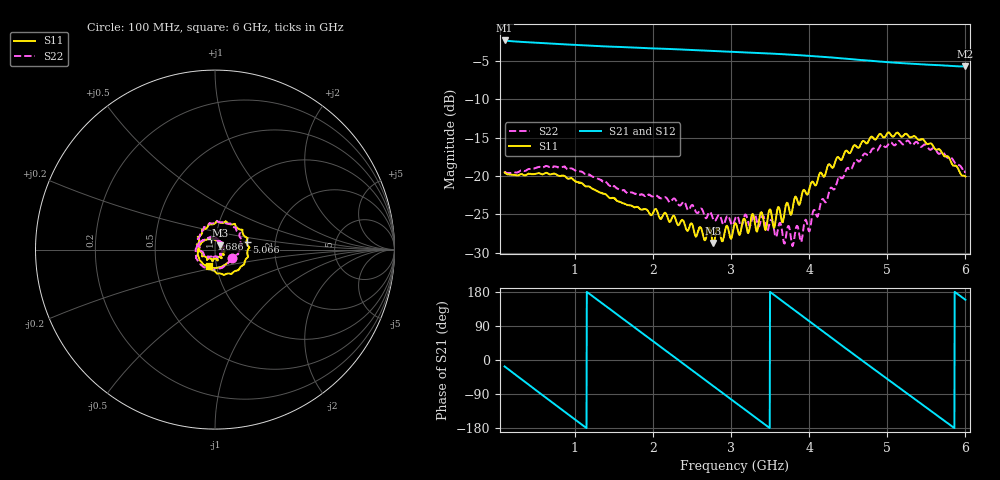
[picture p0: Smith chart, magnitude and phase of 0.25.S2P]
!Agilent Technologies,E5071C,MY46316741,A.11.02
!Date: Thu Dec 16 09:44:38 2021
!Data & Calibration Information:
!Freq	S11:SOLT4(ON)	S21:SOLT4(ON)	S12:SOLT4(ON)	S22:SOLT4(ON)
!PortZ  Port1:50+j0  Port2:50+j0
!Above PortZ is port z conversion or system Z0 setting when saving the data.
!When reading, reference impedance value at option line is always used.
# Hz S dB R 50
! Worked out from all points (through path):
!   1593 points, 100 MHz to 6 GHz, reference 50 ohm
!   highest |S21| = -2.30 dB at 100 MHz (marker M1); lowest = -5.7 dB at 6 GHz (marker M2)
!   group delay of S21, straight-line fit = 426 ps
!   lowest |S11| = -28.7 dB at 2.772 GHz (marker M3), VSWR 1.08, Z = 52.8 + j2.47 ohm
!   |S11| at or under -10 dB: start of sweep to end of sweep
!   |S22| runs from -29.2 to -15.4 dB; largest |S21 - S12| = 0.0046
!   S11 on the Smith chart (normalised r, x): 100 MHz: 1.20, -0.12; 1.686 GHz: 0.95, +0.11; 5.066 GHz: 1.42, +0.12; 6 GHz: 0.92, -0.17
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1e8  -19.53 -27.9  -2.30 -17.0  -2.31 -17.0  -19.41 -27.2
3.631281e8  -19.92 -79.6  -2.52 -58.1  -2.52 -58.1  -19.34 -77.3
5.780779e8  -19.78 -119.2  -2.64 -91.6  -2.65 -91.6  -18.89 -114.7
8.041457e8  -20.00 -156.2  -2.77 -126.6  -2.78 -126.6  -18.87 -148.8
1.085804e9  -20.92 165.5  -2.93 -170.1  -2.93 -170.0  -19.43 177.2
1.36005e9  -22.30 135.5  -3.07 147.9  -3.08 148.0  -20.70 151.8
1.686181e9  -23.81 110.8  -3.20 97.8  -3.21 97.8  -22.26 133.0
2.067902e9  -24.99 88.3  -3.36 39.3  -3.37 39.4  -22.71 112.0
2.405151e9  -26.31 63.0  -3.50 -12.5  -3.51 -12.5  -23.44 91.0
2.772048e9  -28.74 39.8  -3.67 -68.8  -3.69 -68.7  -25.69 74.1
3.05e9  -26.21 16.4  -3.81 -111.4  -3.82 -111.3  -25.66 54.8
3.305716e9  -26.16 -8.3  -3.93 -150.6  -3.94 -150.4  -25.03 39.5
3.528078e9  -25.73 -51.3  -4.03 175.2  -4.03 175.4  -25.92 5.2
3.7875e9  -24.25 -126.0  -4.18 135.2  -4.18 135.4  -29.16 -55.1
4.035804e9  -20.74 -174.6  -4.34 97.0  -4.34 97.2  -25.34 -129.2
4.27299e9  -18.62 142.4  -4.51 60.6  -4.52 60.7  -21.56 -175.5
4.550942e9  -16.44 88.4  -4.75 18.0  -4.75 18.2  -18.90 137.7
5.017902e9  -14.31 19.6  -5.15 -52.8  -5.15 -52.5  -15.77 73.7
5.06608e9  -14.86 13.1  -5.18 -60.0  -5.19 -59.7  -15.78 71.2
5.444095e9  -15.22 -40.8  -5.42 -117.1  -5.42 -116.8  -16.15 24.8
5.72946e9  -17.41 -79.4  -5.58 -160.2  -5.56 -159.8  -17.11 -1.6
6e9  -20.07 -110.8  -5.70 159.0  -5.69 159.3  -19.45 -24.8
